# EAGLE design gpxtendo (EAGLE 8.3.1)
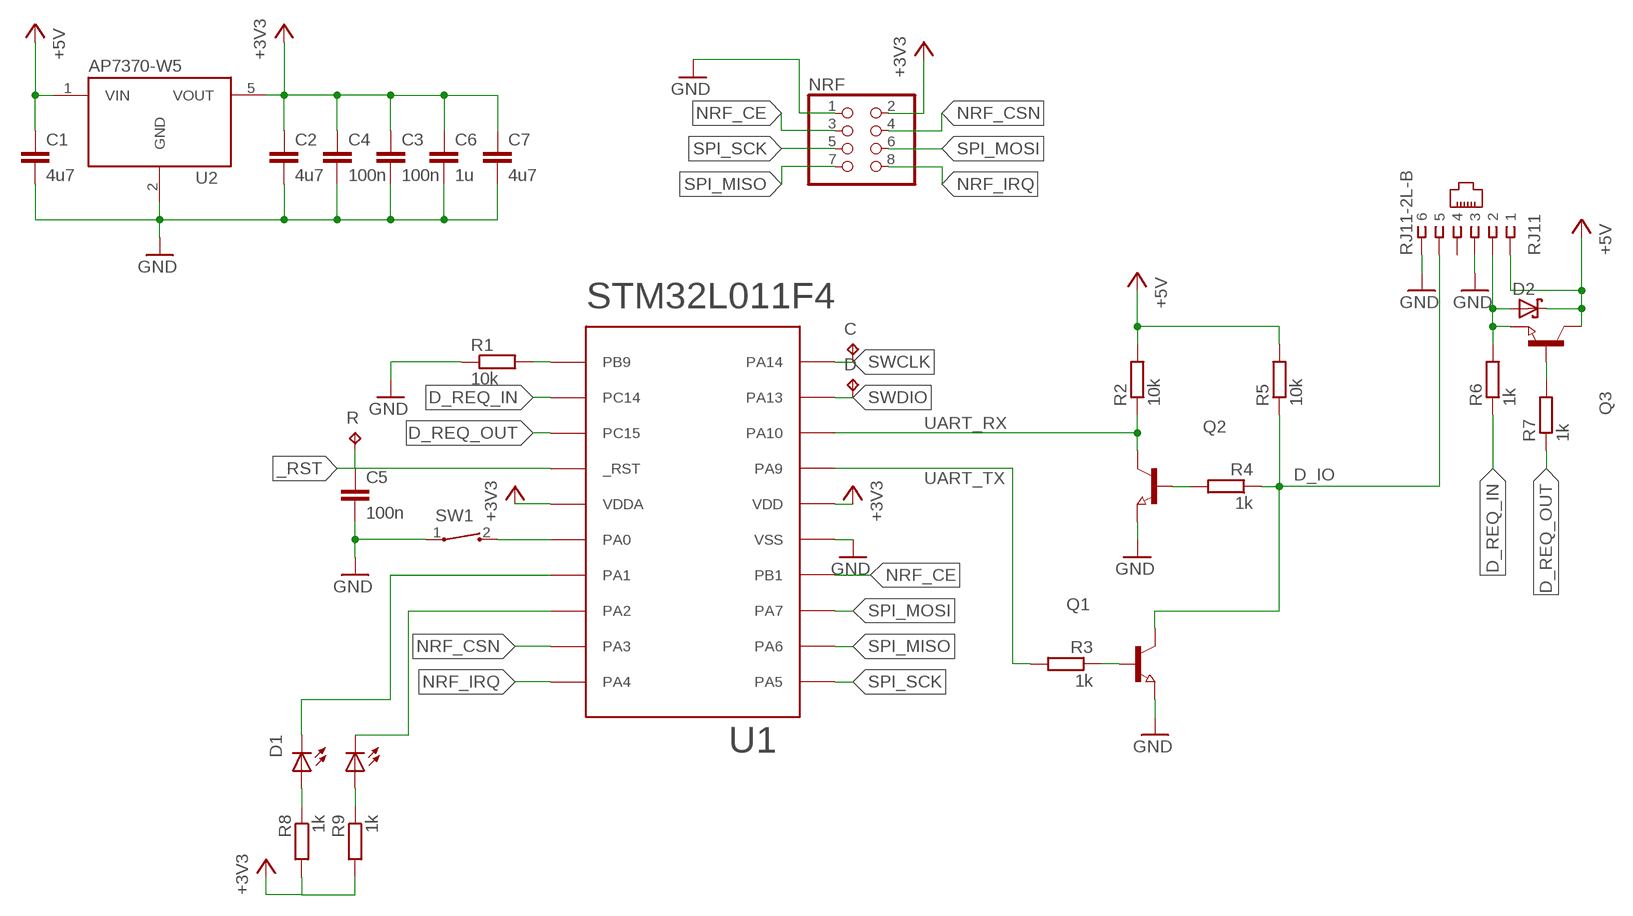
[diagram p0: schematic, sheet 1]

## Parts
C  TPTP10R  [TP10R]
C1  4u7  C0603-S  [C0603-S]
C2  4u7  C0603-S  [C0603-S]
C3  100n  C0603-S  [C0603-S]
C4  100n  C0603-S  [C0603-S]
C5  100n  C0603-S  [C0603-S]
C6  1u  C0603-S  [C0603-S]
C7  4u7  C0603-S  [C0603-S]
D  TPTP10R  [TP10R]
D1  LED-DUAL  [LED-1210]
D2  PMEG4030  [SOD123]
NRF  PINHD-2X4  [2X04]
Q1  NPN-TRANSISTOR_SOT23  [SOT23]
Q2  NPN-TRANSISTOR_SOT23  [SOT23]
Q3  NPN-TRANSISTOR_SOT23  [SOT23]
R  TPTP10R  [TP10R]
R1  10k  R0603-S  [R0603-S]
R2  10k  R0603-S  [R0603-S]
R3  1k  R0603-S  [R0603-S]
R4  1k  R0603-S  [R0603-S]
R5  10k  R0603-S  [R0603-S]
R6  1k  R0603-S  [R0603-S]
R7  1k  R0603-S  [R0603-S]
R8  1k  R0603-S  [R0603-S]
R9  1k  R0603-S  [R0603-S]
RJ11  RJ11-2L-B  [RJ11-NO_SHIELD]
SW1  SW-SPST  [TL3330]
U1  STM32L011F4PX  [TSSOP-20]
U2  AP7370-W5  [SOT23-5]

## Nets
+3V3: C2.1 C3.1 C4.1 C6.1 C7.1 NRF.2 R8.2 R9.2 U1.P$5(VDDA) U1.P$16(VDD) U2.5(VOUT)
+5V: C1.1 D2.C Q3.3(C) R2.2 R5.2 RJ11.1 U2.1(VIN)
_RST: C5.1 R.TP U1.P$4(_RST)
BOOT0: R1.2 U1.P$1(PB9)
D_IO: Q1.3(C) R4.1 R5.1 RJ11.5
D_REQ: D2.A Q3.2(E) R6.2 RJ11.2
D_REQ_IN: R6.1 U1.P$2(PC14)
D_REQ_OUT: R7.1 U1.P$3(PC15)
GND: C1.2 C2.2 C3.2 C4.2 C5.2 C6.2 C7.2 NRF.1 Q1.2(E) Q2.2(E) R1.1 RJ11.3 RJ11.6 SW1.1 U1.P$15(VSS) U2.2(GND)
N$1: Q1.1(B) R3.1
N$2: Q2.1(B) R4.2
N$3: D1.1(C0) U1.P$8(PA2)
N$4: D1.3(C1) U1.P$7(PA1)
N$5: Q3.1(B) R7.2
N$6: D1.2(A0) R9.1
N$7: D1.4(A1) R8.1
N$8: SW1.2 U1.P$6(PA0)
NRF_CE: NRF.3 U1.P$14(PB1)
NRF_CSN: NRF.4 U1.P$9(PA3)
NRF_IRQ: NRF.8 U1.P$10(PA4)
SPI_MISO: NRF.7 U1.P$12(PA6)
SPI_MOSI: NRF.6 U1.P$13(PA7)
SPI_SCK: NRF.5 U1.P$11(PA5)
SWCLK: C.TP U1.P$20(PA14)
SWDIO: D.TP U1.P$19(PA13)
UART_RX: Q2.3(C) R2.1 U1.P$18(PA10)
UART_TX: R3.2 U1.P$17(PA9)
Unconnected: RJ11.4

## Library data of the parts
C D R = testpad:TP: Test pad
C1-C7 = misc:C0603-S
D1 = misc:LED-DUAL
D2 = misc:PMEG4030
NRF = pinhead:PINHD-2X4: PIN HEADER
Q1-Q3 = semicon-smd-ipc:NPN-TRANSISTOR_: NPN TRANSISTOR
R1-R9 = misc:R0603-S
RJ11 = con-tycoelectronics:RJ11: CORCOM Modular RJ Jacks No Shield Source: www.tycoelectronics.com .. ENG_DS_1654001_1099_RJ_L_0507.pdf; MF: TYCO ELECTRONICS; MPN: RJ11-2L-B; OC_FARNELL: unknown; OC_NEWARK: 83F4463
SW1 = misc:SW-SPST
U1 = misc:STM32L011F4
U2 = misc:AP7370

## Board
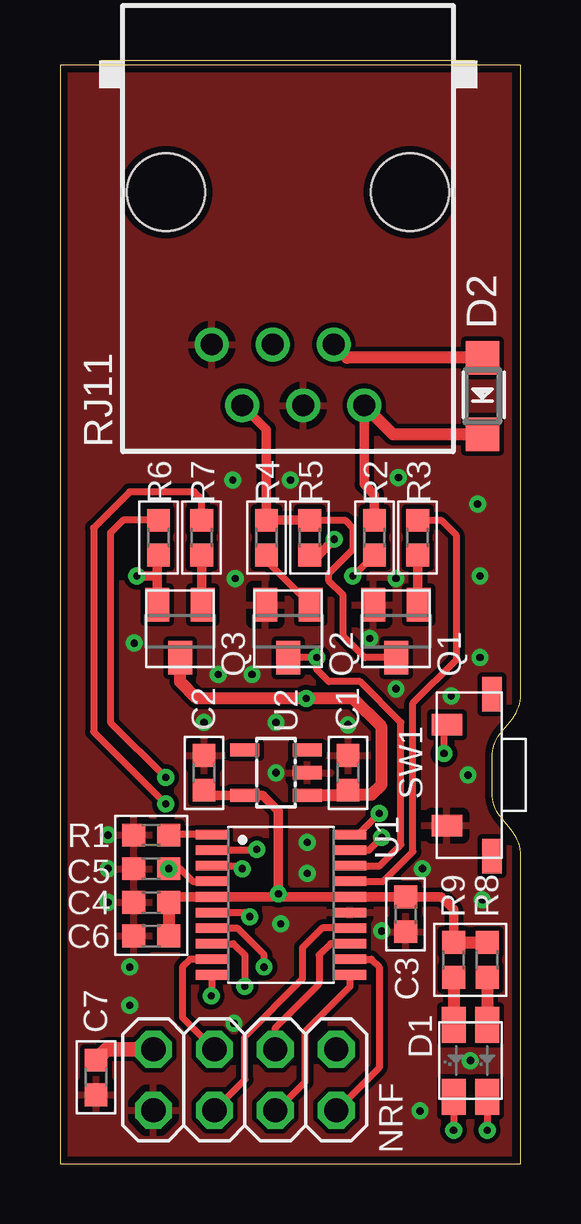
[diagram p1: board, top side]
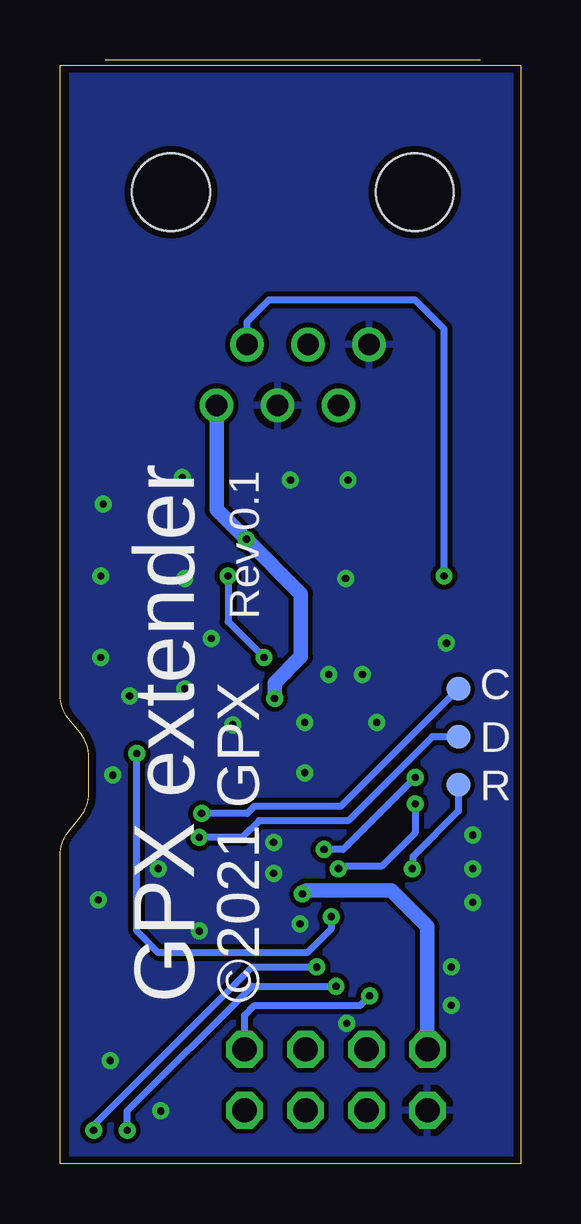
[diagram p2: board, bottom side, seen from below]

Size 19.2 x 46.01 mm. Coordinates in mm from the lower left corner, seen from the top.
Outline: 0,0 19.2,0 19.2,12.85 arc39 18.86,13.83 18.34,14.47 arc-39 18,15.45 18,16.95 arc-39 18.34,17.93 18.86,18.57 arc39 19.2,19.55 19.2,45.8 0,45.8 0,0
Copper layers (1*16): Top 0.035mm / dielectric 1.5mm / Bottom 0.035mm
Design rules "aisler": minimum track width 0.1mm, minimum drill 0.3mm, track to track 0.2mm, track to pad 0.2mm, pad to pad 0.2mm, via to via 0.2mm, smd to smd 0.1mm, copper to edge 0.3mm, drill to drill 6mil, minimum pad ring 10mil, minimum via ring 8mil, stop-mask expansion 0.1mm, vias tented up to drill 99mm, thermal gap 0.3mm

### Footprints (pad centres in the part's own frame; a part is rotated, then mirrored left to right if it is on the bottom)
TP10R = smd 1 x 1: TP 0,0
C0603-S = smd 0.95 x 0.95: 1 -0.725,0; 2 0.725,0
LED-1210 = smd 1.5 x 1: 1 -1.5,0.7; 2 1.5,0.7; 3 -1.5,-0.7; 4 1.5,-0.7
SOD123 = smd 1.4 x 1.4: A 1.6,0; C -1.6,0
2X04 = drill 1.016 octagon: 1 -3.81,-1.27; 2 -3.81,1.27; 3 -1.27,-1.27; 4 -1.27,1.27; 5 1.27,-1.27; 6 1.27,1.27; 7 3.81,-1.27; 8 3.81,1.27
SOT23 = smd 1 x 1.4: 1 -0.95,-1.1; 2 0.95,-1.1; 3 0,1.1
R0603-S = smd 0.95 x 0.95: 1 -0.725,0; 2 0.725,0
RJ11-NO_SHIELD = drill 0.9 pad 1.4: 1 -3.175,8.89; 2 -1.905,6.35; 3 -0.635,8.89; 4 0.635,6.35; 5 1.905,8.89; 6 3.175,6.35 | hole 3.251: -5.08,0; 5.08,0
TL3330 = smd 0.9 x 1.27: 1 -2.1,0.885; 2 2.1,0.885 | smd 1.45 x 0.8: CH0 3.375,-1; CH1 -3.375,-1
TSSOP-20 = smd 0.4 x 1.35: P$1 -2.925,-2.875; P$2 -2.275,-2.875; P$3 -1.625,-2.875; P$4 -0.975,-2.875; P$5 -0.325,-2.875; P$6 0.325,-2.875; P$7 0.975,-2.875; P$8 1.625,-2.875; P$9 2.275,-2.875; P$10 2.925,-2.875; P$11 2.925,2.875; P$12 2.275,2.875; P$13 1.625,2.875; P$14 0.975,2.875; P$15 0.325,2.875; P$16 -0.325,2.875; P$17 -0.975,2.875; P$18 -1.625,2.875; P$19 -2.275,2.875; P$20 -2.925,2.875
SOT23-5 = smd 0.55 x 1.2: 1 -0.95,-1.3; 2 0,-1.3; 3 0.95,-1.3; 4 0.95,1.3; 5 -0.95,1.3

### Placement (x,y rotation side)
C  2.6,19.8 0 bottom
C1  12,16.3 90 top
C2  6,16.3 90 top
C3  14.4,10.4 270 top
C4  3.8,10.9 180 top
C5  3.8,12.3 180 top
C6  3.8,9.5 180 top
C7  1.5,3.6 270 top
D  2.6,17.8 0 bottom
D1  17.1,4.3 90 top
D2  17.6,32 90 top
NRF  7.7,3.5 0 top
Q1  14,22.2 180 top
Q2  9.5,22.2 180 top
Q3  5,22.2 180 top
R  2.6,15.8 0 bottom
R1  3.8,13.7 0 top
R2  13.1,26.1 90 top
R3  14.9,26.1 90 top
R4  8.6,26.1 270 top
R5  10.4,26.1 270 top
R6  4.1,26.1 270 top
R7  5.9,26.1 270 top
R8  17.8,8.5 90 top
R9  16.4,8.5 90 top
RJ11  9.5,40.5 180 top
SW1  17,16.2 90 top
U1  9.2,10.8 270 top
U2  9,16.3 90 top

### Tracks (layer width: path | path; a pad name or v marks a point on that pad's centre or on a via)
+3V3  (via drill 0.3)
  Top 0.3: 4.65,11.12 4.65,11.03 C4.1
  Top 0.4: 4.65,11.12 U1.P$5 8.98,11.12 | C2.1 6.22,15.35 U2.5 8.45,15.35 9.1,14.7 v9.1,11.25 8.98,11.12 | 8.98,11.12 U1.P$16 C3.1 15.88,11.12 16.4,10.6 R9.2
  Top 0.5: C4.1 C6.1 | R9.2 R8.2
  Top 0.6: NRF.2 1.95,4.77 C7.1
  Bottom 0.6: NRF.2 3.89,9.89 5.4,11.4 8.95,11.4 v9.1,11.25
+5V  (via drill 0.3)
  Top 0.4: R5.2 10.78,25.38 v11.43,26.03 | RJ11.1 12.68,28.32 13.1,27.9 R2.2
  Top 0.5: U2.1 11.78,15.35 11.8,15.38 | 11.8,15.38 C1.1 | 11.8,15.38 12.97,15.38 13.4,15.8 13.4,18.2 12.2,19.4 v10.26,19.4 5.7,19.4 5,20.1 Q3.3 | D2.C 13.88,30.4 RJ11.1
  Bottom 0.6: RJ11.1 12.68,27.27 v11.43,26.03 9.16,23.76 9.16,21.14 10.26,20.04 v10.26,19.4
_RST  (via drill 0.3)
  Top 0.3: U1.P$4 5.53,11.78 5,12.3 v4.53,12.3
  Bottom 0.3: R.TP 2.6,14.7 4.5,12.8 4.5,12.32 v4.53,12.3
BOOT0
  Top 0.3: U1.P$1 4.55,13.72 R1.2
D_IO
  Top 0.3: Q1.3 12.7,21.1 11.8,22 11.8,23.7 11.2,24.3 11.2,24.6 12.2,25.6 12.2,26.5 11.88,26.82 R5.1
  Top 0.4: R5.1 R4.1 8.6,30.61 RJ11.5
D_REQ  (via drill 0.3)
  Top 0.3: 4.05,24.5
  Top 0.4: Q3.2 4.05,24.5 | v3.2,24.5 4.05,24.5 | 4.05,24.5 4.05,25.32 R6.2
  Top 0.5: D2.A 11.96,33.6 RJ11.2
  Bottom 0.3: RJ11.2 11.4,35.09 10.5,36 4.4,36 3.2,34.8 v3.2,24.5
D_REQ_IN  (via drill 0.3)
  Top 0.3: U1.P$2 8.18,13.07 v8.2,13.1 | R6.1 2.62,26.82 2.1,26.3 2.1,18.4 v4.4,16.1
  Bottom 0.3: v4.4,16.1 7.4,13.1 v8.2,13.1
D_REQ_OUT  (via drill 0.3)
  Top 0.3: U1.P$3 7.47,12.43 v7.6,12.3 | R7.1 5.9,27.7 5.6,28 2.9,28 1.4,26.5 1.4,18 v4.4,15
  Bottom 0.3: v4.4,15 4.4,13.8 5.8,12.4 7.5,12.4 v7.6,12.3
GND  (via drill 0.3)
  other vias: 9,16.3 2,13.7 2,12.3 2,10.9 2.9,8.2 2.9,6.6 17.4,27.5 17.5,24.5 17.5,21.1 14,19.8 12,18.3 7.3,24.4 6.6,20.4 14,24.4 12.9,21.9 9,18.4 7.2,28.5 9.6,28.5 14.1,28.6 17.1,4.3 13.4,9.7 15,2.2 17,16.2 15.1,12.3 10.3,12.1 10.3,13.4 9.2,10 7.25,5.85 17.6,11 6,18.4 8,20.4 3.1,21.7 16.3,19.5
  pour Top: 0,0 18.7,0 18.7,45.7 0,45.7
  pour Bottom: 18.7,0 0,0 0,45.7 18.7,45.7
N$1
  Top 0.3: 14.9,23.35 Q1.1
  Top 0.4: R3.1 14.9,23.35
N$2
  Top 0.3: R4.2 8.6,25.15 Q2.1
N$3  (via drill 0.3)
  Top 0.3: D1.1 v16.4,1.4 | v7.7,7.4 7.7,8.7 7.22,9.18 U1.P$8
  Bottom 0.3: v16.4,1.4 16.4,2.2 11.2,7.4 v7.7,7.4
N$4  (via drill 0.3)
  Top 0.3: D1.3 v17.8,1.4 | v8.5,8.2 8.5,8.7 7.38,9.82 U1.P$7
  Bottom 0.3: v17.8,1.4 17.8,1.6 11.2,8.2 v8.5,8.2
N$5
  Top 0.3: 5.9,23.35 Q3.1
  Top 0.4: R7.2 5.9,23.35
N$6
  Top 0.5: R9.1 D1.2
N$7
  Top 0.5: R8.1 D1.4
N$8  (via drill 0.3)
  Top 0.3: U1.P$6 7.72,10.47 v7.9,10.3 | v16,17.1 16,18.18 SW1.2
  Bottom 0.3: v7.9,10.3 7.9,9.8 8.9,8.8 15.1,8.8 16,9.7 v16,17.1
NRF_CE
  Top 0.3: NRF.3 7.7,3.5 7.7,5.3 10.1,7.7 10.1,9 10.93,9.82 U1.P$14
NRF_CSN
  Top 0.3: NRF.4 5.1,6.1 5.1,8.2 5.42,8.53 U1.P$9
NRF_IRQ  (via drill 0.3)
  Top 0.3: U1.P$10 6.33,7.03 v6.3,7
  Bottom 0.3: NRF.8 11.51,6.19 11.1,6.6 6.7,6.6 v6.3,7
SPI_MISO
  Top 0.3: NRF.7 11.53,2.23 13.3,4 13.3,8.2 12.97,8.53 U1.P$12
SPI_MOSI
  Top 0.3: NRF.6 8.97,5.67 10.8,7.5 10.8,8.7 11.28,9.18 U1.P$13
SPI_SCK
  Top 0.3: NRF.5 9.03,2.23 10.2,3.4 10.2,5.5 12.07,7.38 U1.P$11
SWCLK  (via drill 0.3)
  Top 0.3: U1.P$20 12.43,13.72 v13.3,14.6
  Bottom 0.3: C.TP 7.5,14.9 11.1,14.9 11.4,14.6 v13.3,14.6
SWDIO  (via drill 0.3)
  Top 0.3: U1.P$19 12.88,13.07 v13.4,13.6
  Bottom 0.3: D.TP 3.7,17.8 7.2,14.3 10.9,14.3 11.6,13.6 v13.4,13.6
UART_RX  (via drill 0.3)
  Top 0.3: 13.07,25.38 R2.1 12.22,24.5 v12.2,24.5 | 10.68,21.1 v10.7,21.1 | 10.68,21.1 Q2.3 | U1.P$18 13.32,12.43 14.2,13.3 14.2,18.4 12.5,20.1 11.2,20.1 10.7,20.6 10.7,21.08 10.68,21.1
  Bottom 0.3: v12.2,24.5 12.2,22.6 v10.7,21.1
UART_TX
  Top 0.3: R3.2 15.88,26.82 16.5,26.2 16.5,21 14.7,19.2 14.7,13 13.47,11.78 U1.P$17

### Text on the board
bPlace: Rev 0.1 | ©2021 GPX | GPX extender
